(* Logix 5000 AddOnInstructionDefinition export Banner_R95C_4B4UI_PD_v4; software revision 33.00 *)

TYPE Banner_R95C_4B4UI_PD_Discrete_v4 :
STRUCT
   P1_DI1 : SINT;
   P1_DI2 : SINT;
   P2_DI1 : SINT;
   P2_DI2 : SINT;
   P3_DI1 : SINT;
   P3_DI2 : SINT;
   P4_DI1 : SINT;
   P4_DI2 : SINT;
   P1_DO1 : SINT;
   P1_DO2 : SINT;
   P2_DO1 : SINT;
   P2_DO2 : SINT;
   P3_DO1 : SINT;
   P3_DO2 : SINT;
   P4_DO1 : SINT;
   P4_DO2 : SINT;
END_STRUCT
END_TYPE

TYPE Banner_R95C_4B4UI_PDI0_v4 :
STRUCT
   Analog_In : DINT[5];
   PDI_Measurement : DINT[5];
   Discrete : Banner_R95C_4B4UI_PD_Discrete_v4;
   Analog_Out : DINT[5];
END_STRUCT
END_TYPE

TYPE Banner_R95C_4B4UI_PDI1_v4 :
STRUCT
   Signal : SINT[4];   // Ports 5 to 8. Indicates the detection status of an object or measurement value within a window.
   Scale : SINT[4];   // Ports 5 to 8.
   Measurement : DINT[9];   // Ports 1 to 8.
   Discrete : Banner_R95C_4B4UI_PD_Discrete_v4;
   Analog_Out : DINT[5];
END_STRUCT
END_TYPE

TYPE Banner_R95C_4B4UI_PDIO_v4 :
STRUCT
   Set0 : Banner_R95C_4B4UI_PDI0_v4;
   Set1 : Banner_R95C_4B4UI_PDI1_v4;
   DTI : SINT[32];
   DTO : SINT[10];
END_STRUCT
END_TYPE

ADD_ON_INSTRUCTION Banner_R95C_4B4UI_PD_v4   (* revision 4.1, vendor Banner Engineering *)
// AOI that used with the R95C-4B4UI-KQ hub.
// Revision note:
// Fixed an issue with Port 2 Discrete 2 ouput not configured correctly.
VAR_IN_OUT
   PD : Banner_R95C_4B4UI_PDIO_v4; {required}
END_VAR
VAR_INPUT
   PDI_Config : SINT; {required}
   Byte_Swap : BOOL; {required}
END_VAR
VAR
   TempIn : SINT[32]; {access None}
   TempOut : SINT[10]; {access None}
END_VAR

ROUTINE Logic   (* ladder *)
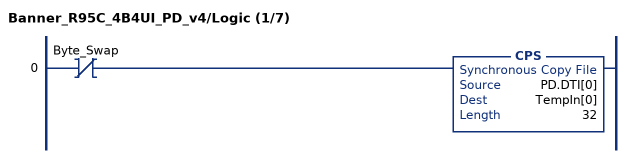
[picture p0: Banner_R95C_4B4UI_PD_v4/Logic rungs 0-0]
   0: XIO(Byte_Swap)CPS(PD.DTI[0],TempIn[0],32);
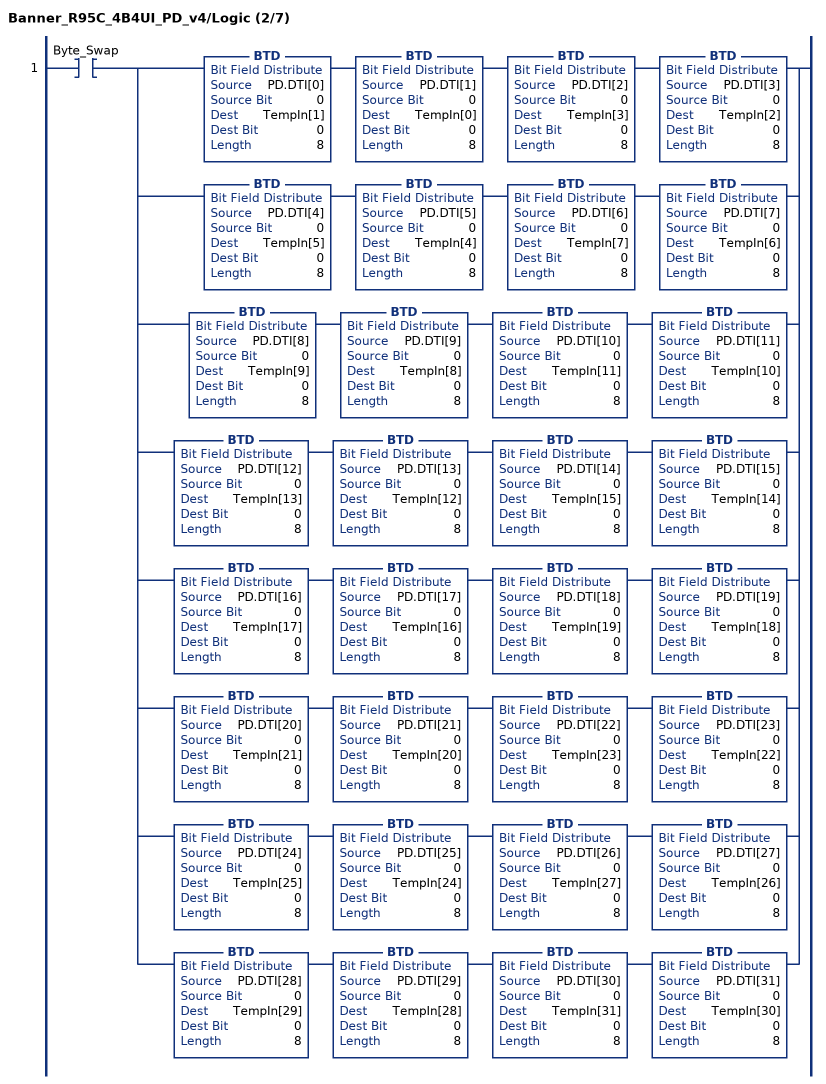
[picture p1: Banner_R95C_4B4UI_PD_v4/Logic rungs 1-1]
   1: XIC(Byte_Swap)[BTD(PD.DTI[0],0,TempIn[1],0,8) BTD(PD.DTI[1],0,TempIn[0],0,8) BTD(PD.DTI[2],0,TempIn[3],0,8) BTD(PD.DTI[3],0,TempIn[2],0,8) ,BTD(PD.DTI[4],0,TempIn[5],0,8) BTD(PD.DTI[5],0,TempIn[4],0,8) BTD(PD.DTI[6],0,TempIn[7],0,8) BTD(PD.DTI[7],0,TempIn[6],0,8) ,BTD(PD.DTI[8],0,TempIn[9],0,8) BTD(PD.DTI[9],0,TempIn[8],0,8) BTD(PD.DTI[10],0,TempIn[11],0,8) BTD(PD.DTI[11],0,TempIn[10],0,8) ,BTD(PD.DTI[12],0,TempIn[13],0,8) BTD(PD.DTI[13],0,TempIn[12],0,8) BTD(PD.DTI[14],0,TempIn[15],0,8) BTD(PD.DTI[15],0,TempIn[14],0,8) ,BTD(PD.DTI[16],0,TempIn[17],0,8) BTD(PD.DTI[17],0,TempIn[16],0,8) BTD(PD.DTI[18],0,TempIn[19],0,8) BTD(PD.DTI[19],0,TempIn[18],0,8) ,BTD(PD.DTI[20],0,TempIn[21],0,8) BTD(PD.DTI[21],0,TempIn[20],0,8) BTD(PD.DTI[22],0,TempIn[23],0,8) BTD(PD.DTI[23],0,TempIn[22],0,8) ,BTD(PD.DTI[24],0,TempIn[25],0,8) BTD(PD.DTI[25],0,TempIn[24],0,8) BTD(PD.DTI[26],0,TempIn[27],0,8) BTD(PD.DTI[27],0,TempIn[26],0,8) ,BTD(PD.DTI[28],0,TempIn[29],0,8) BTD(PD.DTI[29],0,TempIn[28],0,8) BTD(PD.DTI[30],0,TempIn[31],0,8) BTD(PD.DTI[31],0,TempIn[30],0,8) ];
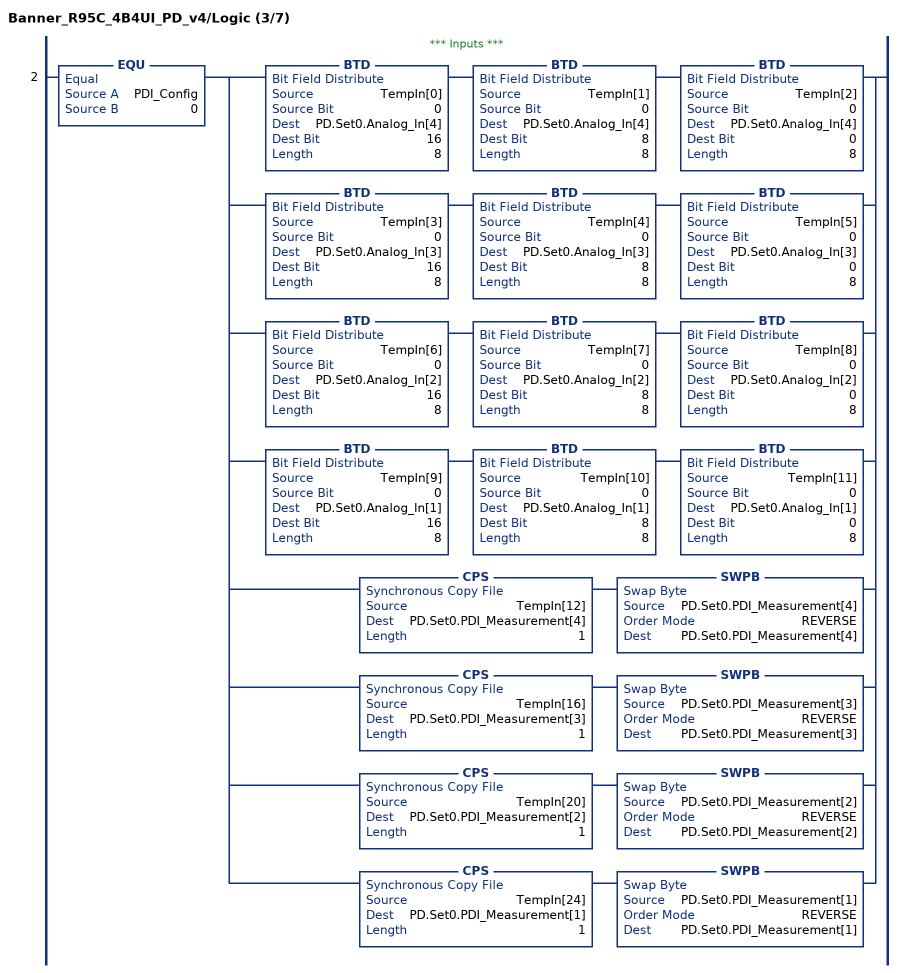
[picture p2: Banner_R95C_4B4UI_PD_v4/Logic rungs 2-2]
   // *** Inputs ***
   2: EQU(PDI_Config,0)[BTD(TempIn[0],0,PD.Set0.Analog_In[4],16,8) BTD(TempIn[1],0,PD.Set0.Analog_In[4],8,8) BTD(TempIn[2],0,PD.Set0.Analog_In[4],0,8) ,BTD(TempIn[3],0,PD.Set0.Analog_In[3],16,8) BTD(TempIn[4],0,PD.Set0.Analog_In[3],8,8) BTD(TempIn[5],0,PD.Set0.Analog_In[3],0,8) ,BTD(TempIn[6],0,PD.Set0.Analog_In[2],16,8) BTD(TempIn[7],0,PD.Set0.Analog_In[2],8,8) BTD(TempIn[8],0,PD.Set0.Analog_In[2],0,8) ,BTD(TempIn[9],0,PD.Set0.Analog_In[1],16,8) BTD(TempIn[10],0,PD.Set0.Analog_In[1],8,8) BTD(TempIn[11],0,PD.Set0.Analog_In[1],0,8) ,CPS(TempIn[12],PD.Set0.PDI_Measurement[4],1) SWPB(PD.Set0.PDI_Measurement[4],REVERSE,PD.Set0.PDI_Measurement[4]) ,CPS(TempIn[16],PD.Set0.PDI_Measurement[3],1) SWPB(PD.Set0.PDI_Measurement[3],REVERSE,PD.Set0.PDI_Measurement[3]) ,CPS(TempIn[20],PD.Set0.PDI_Measurement[2],1) SWPB(PD.Set0.PDI_Measurement[2],REVERSE,PD.Set0.PDI_Measurement[2]) ,CPS(TempIn[24],PD.Set0.PDI_Measurement[1],1) SWPB(PD.Set0.PDI_Measurement[1],REVERSE,PD.Set0.PDI_Measurement[1]) ];
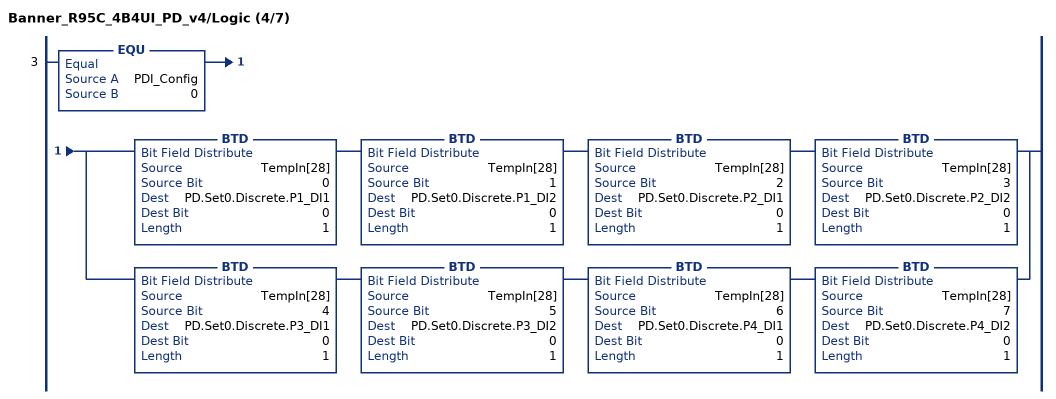
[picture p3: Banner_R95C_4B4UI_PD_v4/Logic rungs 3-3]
   3: EQU(PDI_Config,0)[BTD(TempIn[28],0,PD.Set0.Discrete.P1_DI1,0,1) BTD(TempIn[28],1,PD.Set0.Discrete.P1_DI2,0,1) BTD(TempIn[28],2,PD.Set0.Discrete.P2_DI1,0,1) BTD(TempIn[28],3,PD.Set0.Discrete.P2_DI2,0,1) ,BTD(TempIn[28],4,PD.Set0.Discrete.P3_DI1,0,1) BTD(TempIn[28],5,PD.Set0.Discrete.P3_DI2,0,1) BTD(TempIn[28],6,PD.Set0.Discrete.P4_DI1,0,1) BTD(TempIn[28],7,PD.Set0.Discrete.P4_DI2,0,1) ];
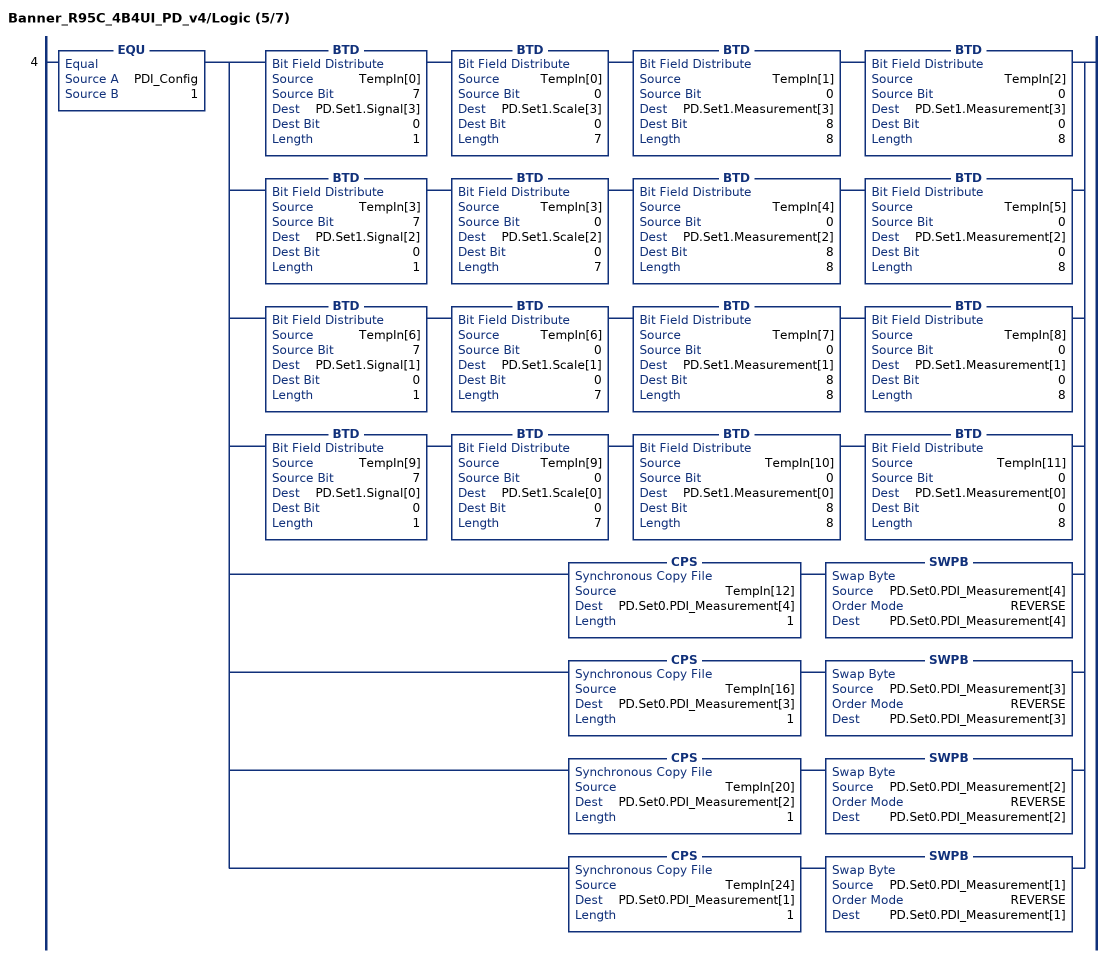
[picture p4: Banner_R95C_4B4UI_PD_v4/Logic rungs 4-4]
   4: EQU(PDI_Config,1)[BTD(TempIn[0],7,PD.Set1.Signal[3],0,1) BTD(TempIn[0],0,PD.Set1.Scale[3],0,7) BTD(TempIn[1],0,PD.Set1.Measurement[3],8,8) BTD(TempIn[2],0,PD.Set1.Measurement[3],0,8) ,BTD(TempIn[3],7,PD.Set1.Signal[2],0,1) BTD(TempIn[3],0,PD.Set1.Scale[2],0,7) BTD(TempIn[4],0,PD.Set1.Measurement[2],8,8) BTD(TempIn[5],0,PD.Set1.Measurement[2],0,8) ,BTD(TempIn[6],7,PD.Set1.Signal[1],0,1) BTD(TempIn[6],0,PD.Set1.Scale[1],0,7) BTD(TempIn[7],0,PD.Set1.Measurement[1],8,8) BTD(TempIn[8],0,PD.Set1.Measurement[1],0,8) ,BTD(TempIn[9],7,PD.Set1.Signal[0],0,1) BTD(TempIn[9],0,PD.Set1.Scale[0],0,7) BTD(TempIn[10],0,PD.Set1.Measurement[0],8,8) BTD(TempIn[11],0,PD.Set1.Measurement[0],0,8) ,CPS(TempIn[12],PD.Set0.PDI_Measurement[4],1) SWPB(PD.Set0.PDI_Measurement[4],REVERSE,PD.Set0.PDI_Measurement[4]) ,CPS(TempIn[16],PD.Set0.PDI_Measurement[3],1) SWPB(PD.Set0.PDI_Measurement[3],REVERSE,PD.Set0.PDI_Measurement[3]) ,CPS(TempIn[20],PD.Set0.PDI_Measurement[2],1) SWPB(PD.Set0.PDI_Measurement[2],REVERSE,PD.Set0.PDI_Measurement[2]) ,CPS(TempIn[24],PD.Set0.PDI_Measurement[1],1) SWPB(PD.Set0.PDI_Measurement[1],REVERSE,PD.Set0.PDI_Measurement[1]) ];
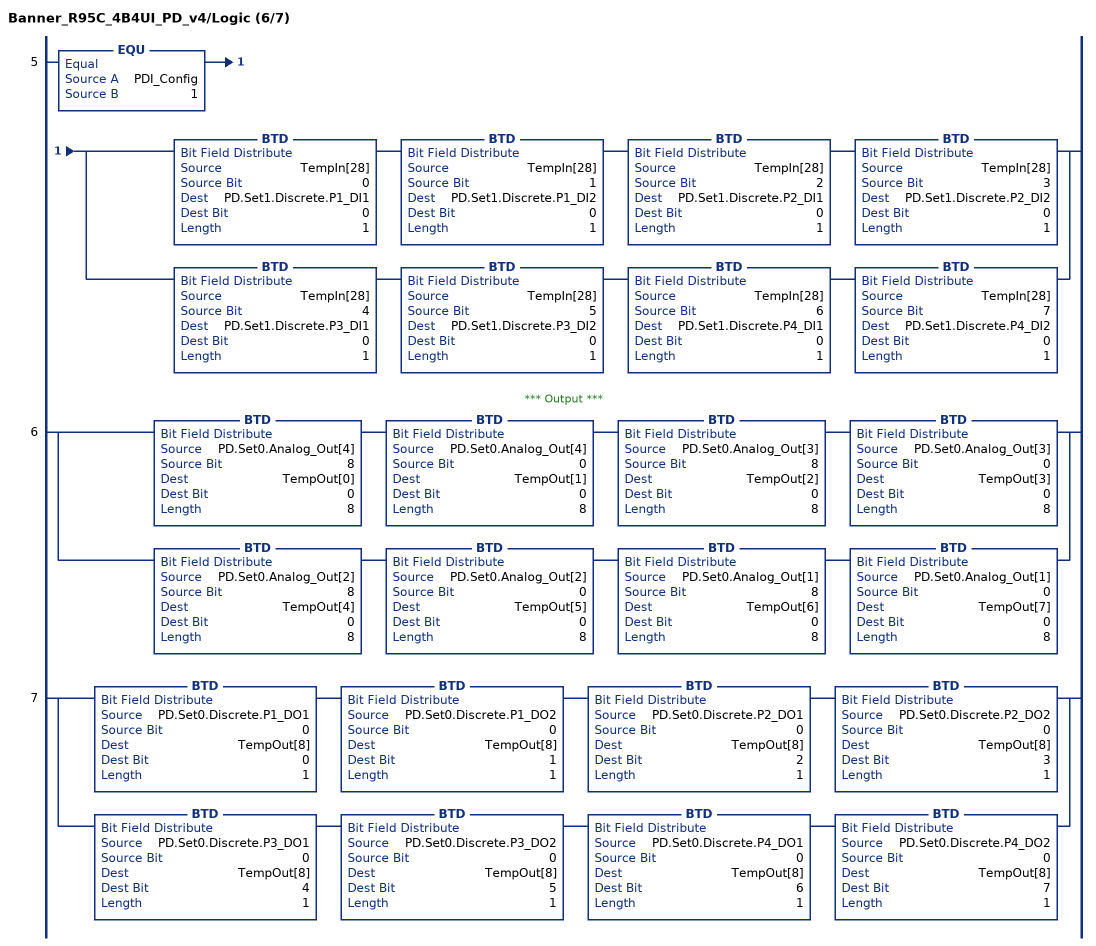
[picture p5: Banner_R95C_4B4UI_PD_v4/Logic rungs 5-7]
   5: EQU(PDI_Config,1)[BTD(TempIn[28],0,PD.Set1.Discrete.P1_DI1,0,1) BTD(TempIn[28],1,PD.Set1.Discrete.P1_DI2,0,1) BTD(TempIn[28],2,PD.Set1.Discrete.P2_DI1,0,1) BTD(TempIn[28],3,PD.Set1.Discrete.P2_DI2,0,1) ,BTD(TempIn[28],4,PD.Set1.Discrete.P3_DI1,0,1) BTD(TempIn[28],5,PD.Set1.Discrete.P3_DI2,0,1) BTD(TempIn[28],6,PD.Set1.Discrete.P4_DI1,0,1) BTD(TempIn[28],7,PD.Set1.Discrete.P4_DI2,0,1) ];
   // *** Output ***
   6: [BTD(PD.Set0.Analog_Out[4],8,TempOut[0],0,8) BTD(PD.Set0.Analog_Out[4],0,TempOut[1],0,8) BTD(PD.Set0.Analog_Out[3],8,TempOut[2],0,8) BTD(PD.Set0.Analog_Out[3],0,TempOut[3],0,8) ,BTD(PD.Set0.Analog_Out[2],8,TempOut[4],0,8) BTD(PD.Set0.Analog_Out[2],0,TempOut[5],0,8) BTD(PD.Set0.Analog_Out[1],8,TempOut[6],0,8) BTD(PD.Set0.Analog_Out[1],0,TempOut[7],0,8) ];
   7: [BTD(PD.Set0.Discrete.P1_DO1,0,TempOut[8],0,1) BTD(PD.Set0.Discrete.P1_DO2,0,TempOut[8],1,1) BTD(PD.Set0.Discrete.P2_DO1,0,TempOut[8],2,1) BTD(PD.Set0.Discrete.P2_DO2,0,TempOut[8],3,1) ,BTD(PD.Set0.Discrete.P3_DO1,0,TempOut[8],4,1) BTD(PD.Set0.Discrete.P3_DO2,0,TempOut[8],5,1) BTD(PD.Set0.Discrete.P4_DO1,0,TempOut[8],6,1) BTD(PD.Set0.Discrete.P4_DO2,0,TempOut[8],7,1) ];
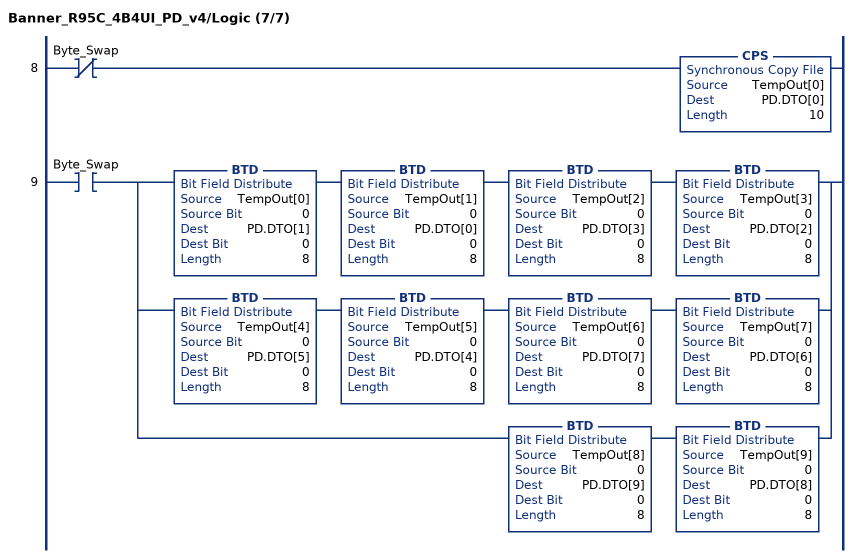
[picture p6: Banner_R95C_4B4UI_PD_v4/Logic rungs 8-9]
   8: XIO(Byte_Swap)CPS(TempOut[0],PD.DTO[0],10);
   9: XIC(Byte_Swap)[BTD(TempOut[0],0,PD.DTO[1],0,8) BTD(TempOut[1],0,PD.DTO[0],0,8) BTD(TempOut[2],0,PD.DTO[3],0,8) BTD(TempOut[3],0,PD.DTO[2],0,8) ,BTD(TempOut[4],0,PD.DTO[5],0,8) BTD(TempOut[5],0,PD.DTO[4],0,8) BTD(TempOut[6],0,PD.DTO[7],0,8) BTD(TempOut[7],0,PD.DTO[6],0,8) ,BTD(TempOut[8],0,PD.DTO[9],0,8) BTD(TempOut[9],0,PD.DTO[8],0,8) ];
END_ROUTINE
END_ADD_ON_INSTRUCTION
